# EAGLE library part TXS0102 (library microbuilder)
2-Bit Bi-Directional Level Shifter (I2C, etc.) Designed for I2C/1-Wire devices and has internal pullups. Not to be confused with TXB010x series. 1.2V-3.6V (VCCA) to 1.65V-5.5V (VCCB) bi-directional level shifter with auto direction sensing. Max data rate - 24Mbps (Push Pull), 2Mbps (Open Drain) Digikey: 296-21931-1-ND NOTE: For cheaper alternative see NXP's NTS0102 (Mouser: 771-NTS0102GT115)
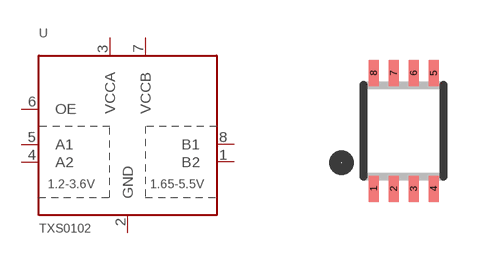
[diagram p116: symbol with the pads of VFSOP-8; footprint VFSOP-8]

Designator prefix U

## TXS0102  [VFSOP-8]
1  B2
2  GND
3  VCCA
4  A2
5  A1
6  OE
7  VCCB
8  B1

## Footprint VFSOP-8 (pad centres in mm)
VFSOP8 - 0.5mm pitch, 2.0x2.3mm Source: http://focus.ti.com/lit/ds/symlink/txs0102.pdf
smd 0.25 x 0.65: 1 -0.75,-1.45; 2 -0.25,-1.45; 3 0.25,-1.45; 4 0.75,-1.45; 5 0.75,1.45; 6 0.25,1.45; 7 -0.25,1.45; 8 -0.75,1.45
